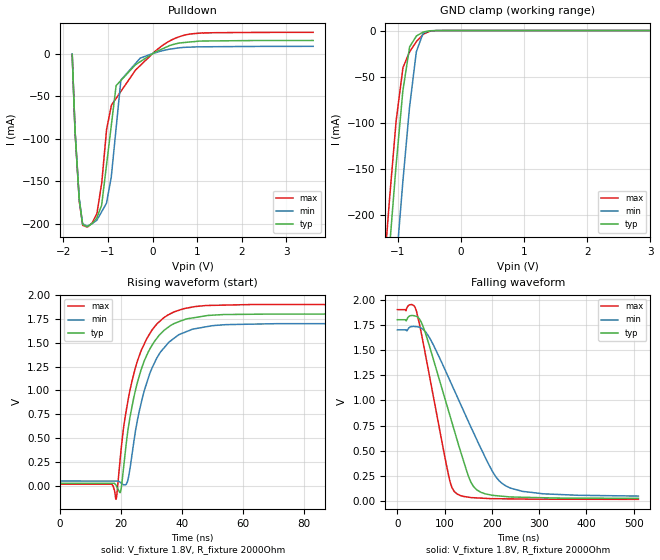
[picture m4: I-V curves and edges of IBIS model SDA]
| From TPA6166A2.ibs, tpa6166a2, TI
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|   SDA
[Model]   SDA
Model_type   I/O_open_drain
Polarity   Non-Inverting
Enable   Active-Low
Vinl = 0.4
Vinh = 1.4
Vmeas = 0.9
Vref = 0.9
Cref = 1pF
Rref = 2000
|   typ   min   max
C_comp   1.8117pF  1.637pF   1.945pF
[Voltage Range]   1.8   1.7   1.9
[Temperature Range]   27   125   -25
[Pullup Reference]   1.8   1.7   1.9
[Pulldown Reference]   -0   -0   -0
[Power Clamp Reference]   1.8   1.7   1.9
[GND Clamp Reference]   -0   -0   -0
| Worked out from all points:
|   slope of the pulldown table from 0 to 0.27 V, typ, clamps not added: 39.4 ohm
|   GND clamp passes 1 mA (typ) near -0.55 V on its own axis
|   falling waveform, V_fixture 1.8V, R_fixture 2000Ohm: 20-80 % time 67.4ns typ, 97.2ns min, 45.8ns max; typ from 1.8 V to 0.029 V
|   rising waveform, V_fixture 1.8V, R_fixture 2000Ohm: 20-80 % time 8.15ns typ, 8.47ns min, 8.09ns max; typ from 0.029 V to 1.8 V
[Pulldown]
|   Voltage   I(typ)   I(min)   I(max)
-1.8V     -657.3uA   -365.1uA   -967.5uA
-1.737V   -90.23mA   -89.87mA   -90.62mA
-1.641V   -171.8mA   -170.7mA   -173.4mA
-1.461V   -203.1mA   -202.3mA   -203.7mA
-1.245V   -192.6mA   -195.2mA   -187.6mA
-1.14V    -177.8mA   -185.5mA   -152.3mA
-1.029V   -129.9mA   -174.6mA   -89mA
-815.8mV  -37.59mA   -87.5mA    -52.53mA
-709mV    -31.55mA   -31.13mA   -44.38mA
-277mV    -9.53mA    -5.385mA   -14.11mA
788.8mV   13.35mA    7.467mA    22.46mA
3.6V      15.42mA    8.508mA    24.95mA
[GND Clamp]
|   Voltage   I(typ)   I(min)   I(max)
-1.8V     -863mA     -973.4mA   -809.4mA
-1.245V   -336.2mA   -448.4mA   -281.8mA
-1.141V   -241.9mA   -353.4mA   -188.9mA
-1.137V   -238.5mA   -349.9mA   -185.4mA
-1.029V   -145.6mA   -254mA     -97.84mA
-921.1mV  -64.7mA    -162.7mA   -40.19mA
-815.8mV  -17.72mA   -82.49mA   -23.13mA
-709mV    -6.043mA   -22.96mA   -12.14mA
-599.8mV  -1.571mA   -2.62mA    -4.124mA
-489.1mV  -253.7uA   -337.9uA   -588.8uA
-381.1mV  -26.99uA   -53.54uA   -40uA
3.6V      0A         0A         0A
[POWER Clamp]
|   Voltage   I(typ)   I(min)   I(max)
-1.8V     0A         0A         0A
0V        0A         0A         0A
3.6V      0A         0A         0A
[Ramp]
R_load = 2000
|   typ   min   max
dV/dt_r   1.06264/8.15583e-009  0.988797/8.46655e-009   1.12836/8.06205e-009
dV/dt_f   1.06269/6.71705e-008  0.988996/9.71727e-008   1.12837/4.57774e-008
[Falling Waveform]
V_fixture = 1.8V
V_fixture_min = 1.7V
V_fixture_max = 1.9V
R_fixture = 2000Ohm
C_fixture = 0F
|   Time   V(typ)   V(min)   V(max)
0s        1.8V       1.7V       1.9V
30.05ns   1.842V     1.732V     1.951V
40.36ns   1.834V     1.731V     1.884V
65.55ns   1.573V     1.64V      1.3V
108.7ns   888.8mV    1.222V     248.8mV
126.6ns   602.7mV    1.035V     71.17mV
161.1ns   146.2mV    680.3mV    35.35mV
200.1ns   59.9mV     304.4mV    26.17mV
229.2ns   46.98mV    152.9mV    24.42mV
510ns     28.84mV    51.63mV    19.38mV
[Rising Waveform]
V_fixture = 1.8V
V_fixture_min = 1.7V
V_fixture_max = 1.9V
R_fixture = 2000Ohm
C_fixture = 0F
|   Time   V(typ)   V(min)   V(max)
0s        28.92mV    51.96mV    19.39mV
16.94ns   28.69mV    51.58mV    18.97mV
18.27ns   10.37mV    51.55mV    -139.6mV
19.82ns   -55.35mV   34.66mV    333.9mV
22.05ns   545.7mV    45.39mV    862.8mV
26.44ns   1.208V     853.7mV    1.409V
29.3ns    1.429V     1.171V     1.591V
32.96ns   1.595V     1.406V     1.734V
44.03ns   1.763V     1.646V     1.878V
510ns     1.8V       1.7V       1.9V
